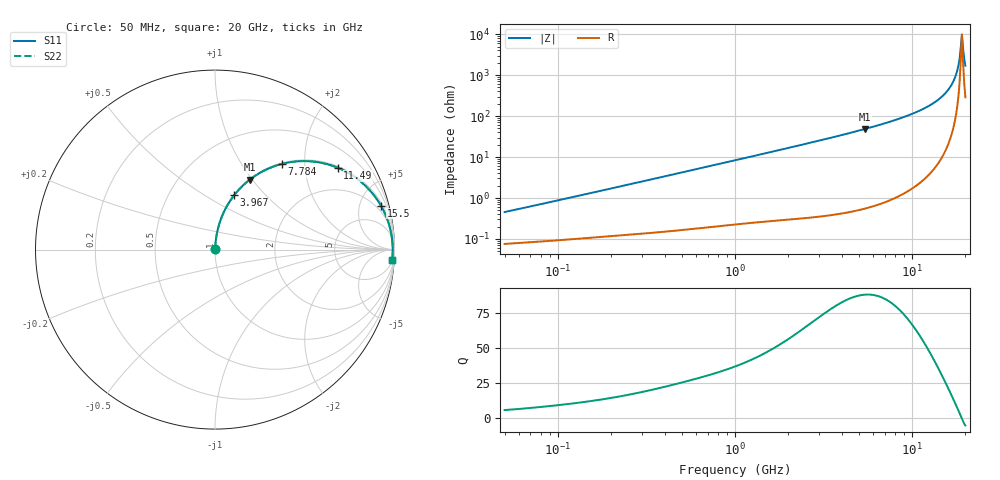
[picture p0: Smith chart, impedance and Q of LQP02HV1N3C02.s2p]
!Murata Part Number: LQP02HV1N3C02
!These Parameters are Measured in Series Mode Connection
!  o--[Z]--o
!Port1  Port2
!  o-------o
!Freq. Start=50[MHz] Stop=20[GHz], 401[Steps]
# Hz S RI R 50
!Freq.(Hz) S11(Real) S11(Imag) S21(Real) S21(Imag) S12(Real) S12(Imag) S22(Real) S22(Imag)
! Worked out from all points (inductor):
!   401 points, 50 MHz to 20 GHz, reference 50 ohm
!   read as one part in series: L = 1.41 nH near 51.52 MHz
!   highest Q = 87.9 at 5.434 GHz (marker M1), where L = 1.43 nH
!   self-resonance near 18.84 GHz
!   S11 on the Smith chart (normalised r, x): 50 MHz: 1.00, +0.01; 3.967 GHz: 1.01, +0.68; 7.784 GHz: 1.02, +1.54; 11.49 GHz: 1.05, +2.96; 15.5 GHz: 1.30, +7.46; 20 GHz: 7, -33
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5e7  0.000777 0.00448  0.9992 -0.00448  0.9992 -0.00448  0.000777 0.00448
1.364002e8  0.00117 0.0118  0.9988 -0.0118  0.9988 -0.0118  0.00117 0.0118
3.721004e8  0.00244 0.0313  0.9976 -0.0313  0.9976 -0.0313  0.00244 0.0313
1e9  0.00912 0.0824  0.9909 -0.0824  0.9909 -0.0824  0.00912 0.0824
2.728004e9  0.0529 0.2167  0.9471 -0.2167  0.9471 -0.2167  0.0529 0.2167
3.967106e9  0.1073 0.3035  0.8927 -0.3035  0.8927 -0.3035  0.1073 0.3035
5.433528e9  0.1942 0.3899  0.8058 -0.3899  0.8058 -0.3899  0.1942 0.3899
7.442007e9  0.3443 0.4692  0.6557 -0.4692  0.6557 -0.4692  0.3443 0.4692
7.784049e9  0.3724 0.4773  0.6276 -0.4773  0.6276 -0.4773  0.3724 0.4773
9.600142e9  0.527 0.4921  0.473 -0.4921  0.473 -0.4921  0.527 0.4921
1.149051e10  0.6837 0.4561  0.3163 -0.4561  0.3163 -0.4561  0.6837 0.4561
1.354865e10  0.8278 0.3651  0.1722 -0.3651  0.1722 -0.3651  0.8278 0.3651
1.550395e10  0.9245 0.245  0.0755 -0.245  0.0755 -0.245  0.9245 0.245
1.670968e10  0.962 0.1629  0.038 -0.1629  0.038 -0.1629  0.962 0.1629
1.747767e10  0.9774 0.1099  0.0226 -0.1099  0.0226 -0.1099  0.9774 0.1099
1.800918e10  0.9844 0.0734  0.0156 -0.0734  0.0156 -0.0734  0.9844 0.0734
1.855685e10  0.9886 0.0364  0.0114 -0.0364  0.0114 -0.0364  0.9886 0.0364
1.88369e10  0.9896 0.0178  0.0104 -0.0178  0.0104 -0.0178  0.9896 0.0178
1.912117e10  0.99 -0.00092  0.01 0.00092  0.01 0.00092  0.99 -0.00092
1.940974e10  0.9896 -0.0196  0.0104 0.0196  0.0104 0.0196  0.9896 -0.0196
1.970266e10  0.9886 -0.0382  0.0114 0.0382  0.0114 0.0382  0.9886 -0.0382
2e10  0.9868 -0.0568  0.0132 0.0568  0.0132 0.0568  0.9868 -0.0568
